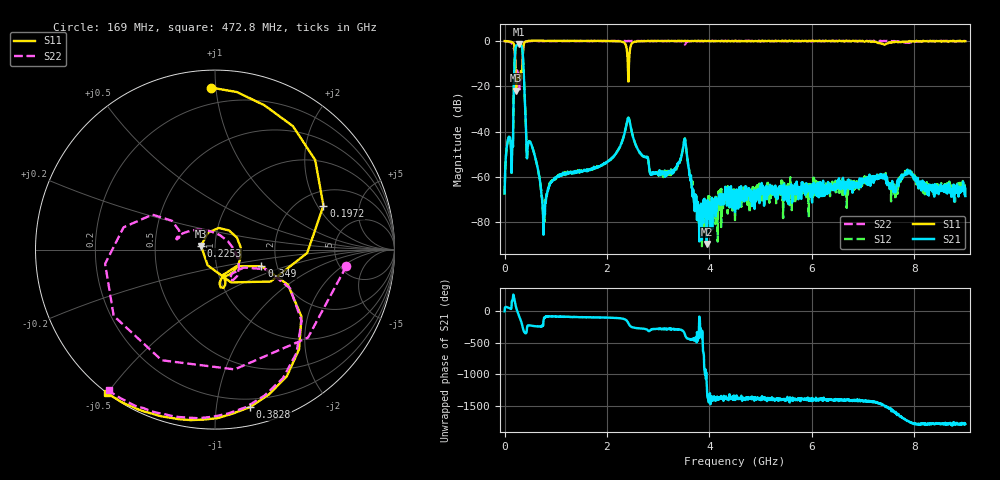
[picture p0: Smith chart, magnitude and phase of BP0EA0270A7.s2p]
!Agilent Technologies,E8358A,US40260310,A.06.04.32
!Agilent E8358A: A.06.04.32
!Date: Sunday, April 05, 2020 20:55:32
!Correction: S11(Full 2 Port(1,2)) S21(Full 2 Port(1,2)) S12(Full 2 Port(1,2)) S22(Full 2 Port(1,2))
!S2P File: Measurements: S11, S21, S12, S22:
# Hz S  dB  R 50
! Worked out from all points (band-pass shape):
!   1601 points, 300 kHz to 9 GHz, reference 50 ohm
!   highest |S21| = -1.57 dB at 281.5 MHz (marker M1); lowest = -89.6 dB at 3.949 GHz (marker M2)
!   |S21| within 3 dB of the highest: 207.1 MHz to 351 MHz (143.9 MHz wide, 51.6 % of centre)
!   lowest |S11| = -21.9 dB at 225.3 MHz (marker M3), VSWR 1.17, Z = 42.8 + j1.72 ohm
!   |S11| at or under -10 dB: 209.6 MHz to 350.6 MHz (141 MHz wide, 50.3 % of centre); 2.406 GHz to 2.429 GHz (23.16 MHz wide, 0.958 % of centre)
!   |S22| runs from -21.4 to 0.1 dB; largest |S21 - S12| = 0.0074
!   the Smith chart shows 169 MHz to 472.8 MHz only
!   S11 on the Smith chart (normalised r, x): 169 MHz: 0.10, +0.97; 197.2 MHz: 2.66, +2.26; 225.3 MHz: 0.86, +0.03; 349 MHz: 1.66, -0.33; 382.8 MHz: 0.14, -1.24; 472.8 MHz: 0.00, -0.50
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300000  -0.09 179.9  -67.29 2.6  -67.92 -1.8  -0.18 180.0
1.127962e8  -0.33 139.9  -43.78 44.9  -43.62 44.4  -0.56 129.5
1.690444e8  -0.89 91.3  -35.52 -90.4  -35.50 -90.6  -2.64 -7.1
1.971684e8  -3.72 22.0  -8.40 174.7  -8.41 174.4  -4.19 -172.6
2.252925e8  -21.91 165.6  -2.10 62.9  -2.09 62.7  -13.54 161.1
2.815406e8  -15.92 -69.5  -1.57 -67.6  -1.55 -67.8  -17.94 119.0
3.490384e8  -11.23 -19.7  -4.02 123.9  -3.99 124.1  -10.37 -21.1
3.827872e8  -0.93 -77.4  -18.94 33.9  -18.90 34.1  -0.97 -78.8
4.727842e8  -0.01 -127.1  -44.46 140.3  -44.49 140.2  -0.16 -127.1
7.652745e8  -0.04 -161.8  -80.22 -131.9  -78.74 -136.2  -0.08 -158.4
1.502125e9  -0.03 178.4  -57.42 -88.6  -57.42 -91.7  -0.06 -175.5
2.250225e9  -0.25 161.9  -46.80 -107.9  -46.82 -108.0  -0.15 173.8
2.418969e9  -17.99 -19.3  -33.95 171.1  -33.88 170.8  -0.06 171.0
2.54834e9  -0.35 -167.4  -45.27 97.6  -45.14 97.0  -0.05 169.3
3.00395e9  -0.01 177.5  -59.22 80.1  -57.62 81.3  -0.04 163.2
3.515808e9  -0.01 172.9  -43.17 6.0  -43.36 7.6  -1.51 154.9
3.808298e9  -0.08 168.7  -75.29 172.2  -83.35 -158.4  -0.11 154.5
3.948918e9  -0.14 167.2  -89.60 -100.4  -72.28 127.9  -0.16 153.3
4.50015e9  0.02 156.4  -75.54 28.9  -79.10 79.8  -0.04 152.0
6.001975e9  0.10 140.1  -70.95 10.5  -63.39 32.6  -0.17 131.7
7.5038e9  -0.83 139.2  -63.63 -107.0  -63.09 -115.6  -0.15 123.9
9e9  -0.14 122.2  -68.48 8.4  -64.21 -4.6  -0.11 124.8
